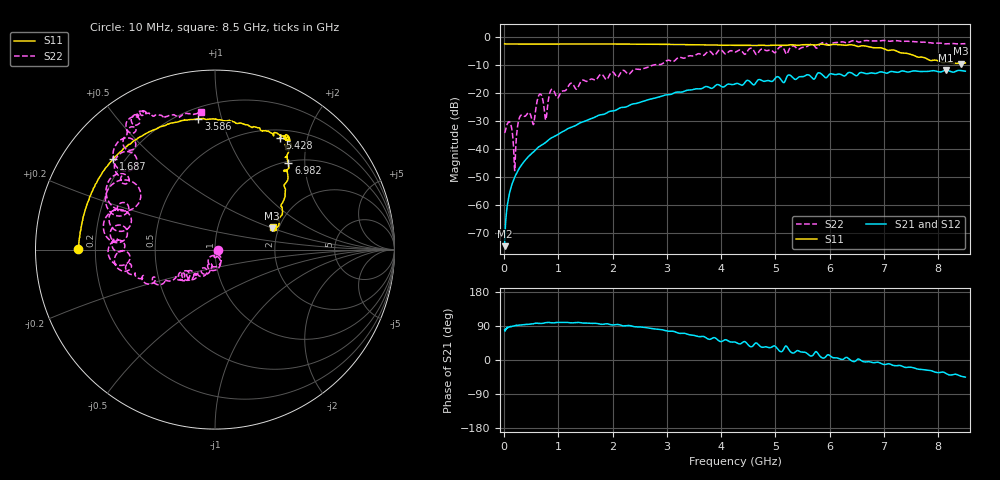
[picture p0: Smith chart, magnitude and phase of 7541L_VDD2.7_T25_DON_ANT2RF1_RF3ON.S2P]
!Agilent Technologies,E5071C,MY46417908,A.11.23
!Date: Wed Dec 09 17:17:54 2020
!Data & Calibration Information:
!Freq	S11:SOLT2(ON)	S21:SOLT2(ON)	S12:SOLT2(ON)	S22:SOLT2(ON)
!PortZ  Port1:50+j0  Port2:50+j0
!Above PortZ is port z conversion or system Z0 setting when saving the data.
!When reading, reference impedance value at option line is always used.
# Hz S dB R 50
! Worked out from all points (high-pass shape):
!   1601 points, 10 MHz to 8.5 GHz, reference 50 ohm
!   highest |S21| = -11.75 dB at 8.144 GHz (marker M1); lowest = -74.9 dB at 10 MHz (marker M2)
!   |S21| within 3 dB of the highest: 5.4 GHz to 5.686 GHz (286.2 MHz wide, 5.16 % of centre); 5.727 GHz to end of sweep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
!   lowest |S11| = -9.5 dB at 8.42 GHz (marker M3), VSWR 2.01, Z = 91.7 + j24.4 ohm
!   |S11| at or under -10 dB: nowhere
!   |S22| runs from -47.8 to -1.1 dB; largest |S21 - S12| = 0.0029
!   S11 on the Smith chart (normalised r, x): 10 MHz: 0.13, +0.00; 1.687 GHz: 0.16, +0.37; 3.586 GHz: 0.27, +0.85; 5.428 GHz: 0.61, +1.57; 6.982 GHz: 1.04, +1.66; 8.5 GHz: 1.86, +0.53
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1e7  -2.33 179.6  -74.89 79.9  -73.81 65.2  -34.30 0.1
1.055125e8  -2.39 177.0  -55.47 87.5  -55.58 86.7  -30.43 -58.8
1.957188e8  -2.41 174.5  -50.22 90.5  -50.25 90.3  -47.79 -52.7
2.700062e8  -2.41 172.5  -47.32 92.2  -47.29 92.0  -29.70 -32.0
3.124562e8  -2.44 171.3  -46.00 92.4  -46.09 92.6  -27.95 -58.4
5.300125e8  -2.42 165.8  -41.33 95.6  -41.31 95.7  -31.00 -87.4
6.573625e8  -2.43 162.5  -39.07 96.6  -39.03 96.6  -20.38 -88.6
7.687938e8  -2.43 159.8  -37.66 98.6  -37.65 98.7  -29.65 -94.5
8.749188e8  -2.42 157.0  -36.04 98.1  -36.07 98.2  -18.69 -92.4
9.916562e8  -2.41 153.9  -34.86 99.2  -34.85 99.2  -21.69 -105.4
1.426769e9  -2.38 144.2  -30.46 97.9  -30.46 97.9  -15.58 -115.7
1.686775e9  -2.39 138.3  -28.50 96.8  -28.50 96.8  -15.31 -126.8
2.843538e9  -2.54 113.0  -21.48 81.0  -21.48 81.0  -9.79 -149.4
3.586412e9  -2.67 97.2  -18.49 61.7  -18.49 61.7  -5.87 -167.7
4.255e9  -2.88 81.1  -16.72 47.3  -16.72 47.3  -5.27 174.3
5.427681e9  -2.86 59.7  -14.29 24.1  -14.26 24.0  -4.26 142.8
5.671769e9  -2.69 57.4  -14.46 10.8  -14.40 10.6  -2.47 135.1
6.982412e9  -3.99 49.6  -12.49 -11.3  -12.50 -11.0  -1.14 119.3
7.088538e9  -4.71 48.8  -12.57 -9.8  -12.63 -9.8  -1.38 117.7
8.144481e9  -8.95 20.5  -11.75 -35.7  -11.78 -35.6  -2.34 105.0
8.420406e9  -9.47 20.6  -11.93 -42.8  -11.99 -42.9  -2.34 97.9
8.5e9  -9.18 21.1  -12.15 -45.2  -12.23 -45.1  -2.26 95.9
